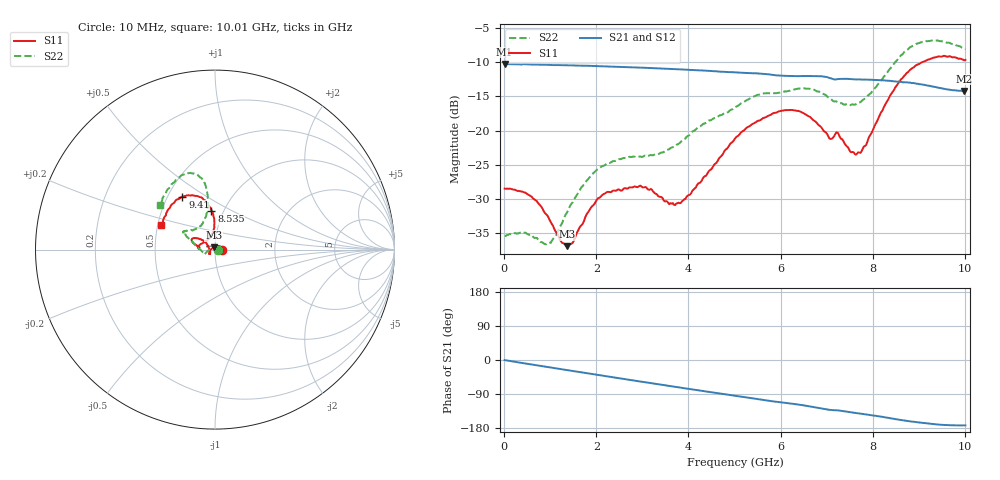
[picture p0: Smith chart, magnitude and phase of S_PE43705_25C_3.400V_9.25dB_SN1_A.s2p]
! Device ID: PE43705
! Serial: 1
! Insertion: A
! Impedance: 50 ohm
! Temp: 25C
! VDD: 3.400V
! Attenuation Step: 9.25dB
#  Hz  S  RI  R  50
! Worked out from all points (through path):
!   401 points, 10 MHz to 10.01 GHz, reference 50 ohm
!   highest |S21| = -10.28 dB at 10 MHz (marker M1); lowest = -14.2 dB at 9.985 GHz (marker M2)
!   group delay of S21, straight-line fit = 49.7 ps
!   lowest |S11| = -36.9 dB at 1.36 GHz (marker M3), VSWR 1.03, Z = 49.3 + j1.22 ohm
!   |S11| at or under -10 dB: start of sweep to 9.078 GHz
!   |S22| runs from -36.6 to -6.8 dB; largest |S21 - S12| = 0.0031
!   S11 on the Smith chart (normalised r, x): 10 MHz: 1.08, +0.00; 8.535 GHz: 0.88, +0.40; 9.41 GHz: 0.59, +0.40; 10.01 GHz: 0.52, +0.16
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1e7  0.0377 0.000129  0.3063 -0.00134  0.3065 -0.00134  0.017 0.000262
5.35e8  0.0291 0.0175  0.2984 -0.0563  0.2985 -0.0561  0.0103 0.014
9.6e8  0.0113 0.0203  0.2855 -0.0976  0.2856 -0.0975  -0.00627 0.0137
1.36e9  -0.00718 0.0124  0.2682 -0.1337  0.2683 -0.1335  -0.0246 0.00466
1.685e9  -0.0204 0.00178  0.2505 -0.1607  0.2506 -0.1607  -0.0385 -0.00548
2.21e9  -0.0313 -0.016  0.2163 -0.1994  0.2165 -0.1993  -0.0529 -0.0207
2.96e9  -0.0308 -0.0249  0.1573 -0.2414  0.1576 -0.2411  -0.0613 -0.0205
3.36e9  -0.0268 -0.0193  0.1233 -0.2561  0.1237 -0.2559  -0.0658 -0.0157
3.635e9  -0.0279 -0.00921  0.0993 -0.2636  0.0994 -0.2635  -0.0747 -0.00835
3.885e9  -0.0309 0.00181  0.0768 -0.2681  0.0772 -0.2678  -0.0846 0.00172
5.01e9  -0.0694 0.0533  -0.0201 -0.2651  -0.0197 -0.2652  -0.1379 0.0541
5.985e9  -0.1237 0.0629  -0.092 -0.2348  -0.0907 -0.235  -0.1663 0.0904
6.685e9  -0.1167 0.033  -0.1371 -0.209  -0.1373 -0.2085  -0.1697 0.1028
7.06e9  -0.0865 0.0132  -0.1602 -0.1811  -0.16 -0.1822  -0.1332 0.1097
7.235e9  -0.0951 0.0185  -0.1615 -0.1741  -0.161 -0.1742  -0.1172 0.1109
7.685e9  -0.0384 0.0578  -0.1827 -0.1503  -0.1826 -0.1499  -0.0735 0.1419
8.36e9  -0.00521 0.1758  -0.2061 -0.1042  -0.205 -0.1053  -0.0393 0.2765
8.535e9  -0.0196 0.2163  -0.2089 -0.09  -0.2074 -0.0919  -0.0455 0.3257
8.935e9  -0.0728 0.2897  -0.2121 -0.0613  -0.211 -0.06  -0.0993 0.4165
9.41e9  -0.1819 0.2947  -0.2033 -0.0349  -0.2026 -0.0347  -0.1861 0.4148
9.985e9  -0.2912 0.1451  -0.1929 -0.0251  -0.1939 -0.0259  -0.2998 0.2576
1.001e10  -0.2982 0.1362  -0.1939 -0.0255  -0.1944 -0.0266  -0.3072 0.2473
